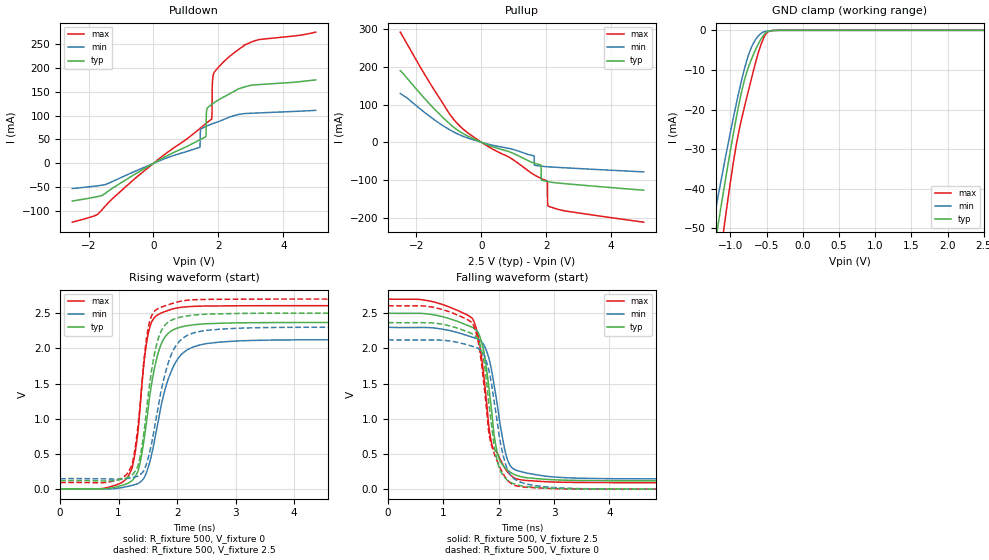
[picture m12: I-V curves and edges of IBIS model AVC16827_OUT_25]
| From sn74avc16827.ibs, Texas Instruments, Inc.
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[Model]   AVC16827_OUT_25
Model_type  3-state
Enable   Active-Low
Vref =   0
Rref =   500
Cref =   30p
Vmeas =   1.25
| variable   typ   min   max
C_comp   4.24pF   3.31pF   5.17pF
| C_pullup   7.99pF   0.72pF   28.19pF
| C_pulldown   15.16pF   2.36pF   45.68pF
| C_tri-state   4.24pF   3.31pF   5.17pF
[Temperature Range]   40   100   -40
| Ambient temperature   25   85   -40
[Voltage range]   2.5   2.3   2.7
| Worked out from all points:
|   slope of the pulldown table from 0 to 0.375 V, typ, clamps not added: 26.1 ohm
|   slope of the pullup table from 0 to 0.375 V, typ, clamps not added: 30.1 ohm
|   GND clamp passes 1 mA (typ) near -0.53 V on its own axis
|   rising waveform, R_fixture 500, V_fixture 0: 20-80 % time 273ps typ, 368ps min, 197ps max; typ from 0 V to 2.37 V
|   falling waveform, R_fixture 500, V_fixture 2.5: 20-80 % time 242ps typ, 286ps min, 255ps max; typ from 2.5 V to 0.119 V
|   rising waveform, R_fixture 500, V_fixture 2.5: 20-80 % time 245ps typ, 336ps min, 197ps max; typ from 0.119 V to 2.5 V
|   falling waveform, R_fixture 500, V_fixture 0: 20-80 % time 237ps typ, 280ps min, 279ps max; typ from 2.37 V to 0 V
[GND Clamp]
| AVC16827_OUT_25
|   Voltage   I(typ)   I(min)   I(max)
-2.5V     -213.6mA   -184mA     -260.4mA
-1.26V    -59.39mA   -50.76mA   -73.5mA
-1.225V   -55.32mA   -47.25mA   -68.55mA
-1.165V   -48.43mA   -41.32mA   -60.17mA
-1.085V   -39.44mA   -33.58mA   -49.27mA
-930mV    -23.12mA   -19.44mA   -30.02mA
-815mV    -13.17mA   -10.31mA   -19.97mA
-695mV    -6.608mA   -3.691mA   -11.11mA
-560mV    -1.681mA   -559uA     -2.73mA
-490mV    -345.1uA   -179.7uA   -514.2uA
-405mV    -36.97uA   -42.08uA   -30.82uA
2.5V      972.5pA    11.08nA    39.96pA
[Pulldown]
| AVC16827_OUT_25
|   Voltage   I(typ)   I(min)   I(max)
-2.5V     -78.94mA   -52.82mA   -123.3mA
-1.73V    -69.72mA   -47.06mA   -107.3mA
1.425V    49.25mA    33.56mA    72.74mA
1.455V    50.31mA    71.5mA     74.42mA
1.61V     55.57mA    77.18mA    83.1mA
1.64V     111.7mA    78.11mA    84.76mA
1.79V     123.3mA    82.33mA    92.64mA
1.805V    124mA      82.7mA     107mA
1.815V    124.5mA    82.95mA    168mA
1.855V    126.5mA    83.88mA    188.1mA
2.485V    151mA      100mA      231.6mA
5V        174.9mA    111.1mA    275.1mA
[Pullup]
| AVC16827_OUT_25
|   Voltage   I(typ)   I(min)   I(max)
-2.5V     189.8mA    129.5mA    292.1mA
-835mV    38.73mA    26.58mA    58.78mA
1.62V     -54.9mA    -35.73mA   -85.82mA
1.635V    -55.33mA   -60.76mA   -86.58mA
1.83V     -60.18mA   -63.23mA   -95.41mA
1.84V     -61.44mA   -63.34mA   -95.82mA
1.85V     -100mA     -63.44mA   -96.22mA
2.025V    -103.7mA   -64.84mA   -102.8mA
2.035V    -103.9mA   -64.9mA    -106.3mA
2.04V     -104mA     -64.93mA   -160.9mA
2.06V     -104.3mA   -65.04mA   -169.3mA
5V        -127mA     -78.45mA   -211.8mA
[Ramp]
| AVC16827_OUT_25
| variable   typ   min   max
dV/dt_r   1.42/2.82E-10   1.27/3.73E-10   1.56/2.06E-10
dV/dt_f   1.43/2.50E-10   1.29/2.86E-10   1.56/2.57E-10
R_load = 500
[Rising Waveform]
| AVC16827_OUT_25
R_fixture =   500
C_fixture =   0
L_fixture =   0
V_fixture =   0
V_fixture_min = 0
V_fixture_max = 0
|   Time   V(typ)   V(min)   V(max)
0s        21.86nV    92.03nV    966.7pV
1.14ns    76.22mV    36.3mV     154.5mV
1.245ns   135.1mV    57.3mV     351.1mV
1.345ns   296.9mV    86.31mV    938.3mV
1.445ns   758.7mV    176.7mV    1.874V
1.545ns   1.392V     425.3mV    2.331V
1.765ns   2.124V     1.321V     2.514V
1.96ns    2.273V     1.78V      2.566V
2.185ns   2.323V     1.984V     2.592V
50ns      2.367V     2.122V     2.606V
[Falling Waveform]
| AVC16827_OUT_25
R_fixture =   500
C_fixture =   0
L_fixture =   0
V_fixture =   2.5
V_fixture_min = 2.3
V_fixture_max = 2.7
|   Time   V(typ)   V(min)   V(max)
0s        2.5V       2.3V       2.7V
1.525ns   2.298V     2.158V     2.425V
1.625ns   2.23V      2.133V     2.188V
1.72ns    2V         2.066V     1.683V
1.82ns    1.456V     1.867V     901.7mV
1.885ns   1.01V      1.627V     605.3mV
1.99ns    471.9mV    1.112V     483.5mV
2.155ns   273.9mV    426.9mV    249.4mV
2.5ns     161.9mV    229.3mV    122.1mV
50ns      118.7mV    145.8mV    92.52mV
[Rising Waveform]
| AVC16827_OUT_25
R_fixture =   500
C_fixture =   0
L_fixture =   0
V_fixture =   2.5
V_fixture_min = 2.3
V_fixture_max = 2.7
|   Time   V(typ)   V(min)   V(max)
0s        118.7mV    145.8mV    92.52mV
990ps     129.8mV    142.5mV    135.3mV
1.255ns   224mV      168.5mV    448.2mV
1.385ns   540.2mV    218.6mV    1.353V
1.465ns   1.027V     330.8mV    2.061V
1.55ns    1.608V     596.6mV    2.433V
1.685ns   2.157V     1.202V     2.57V
1.87ns    2.384V     1.844V     2.625V
2.25ns    2.469V     2.21V      2.689V
50ns      2.5V       2.3V       2.7V
[Falling Waveform]
| AVC16827_OUT_25
R_fixture =   500
C_fixture =   0
L_fixture =   0
V_fixture =   0
V_fixture_min = 0
V_fixture_max = 0
|   Time   V(typ)   V(min)   V(max)
0s        2.367V     2.122V     2.606V
1.525ns   2.205V     2.029V     2.361V
1.625ns   2.131V     2.002V     2.116V
1.72ns    1.876V     1.924V     1.573V
1.82ns    1.232V     1.694V     811.9mV
1.905ns   693.8mV    1.313V     535.4mV
2ns       326.4mV    810mV      347.1mV
2.145ns   135.2mV    308.1mV    140.8mV
2.5ns     35.65mV    72.52mV    26.22mV
50ns      19.74nV    125.5nV    -1.607nV
